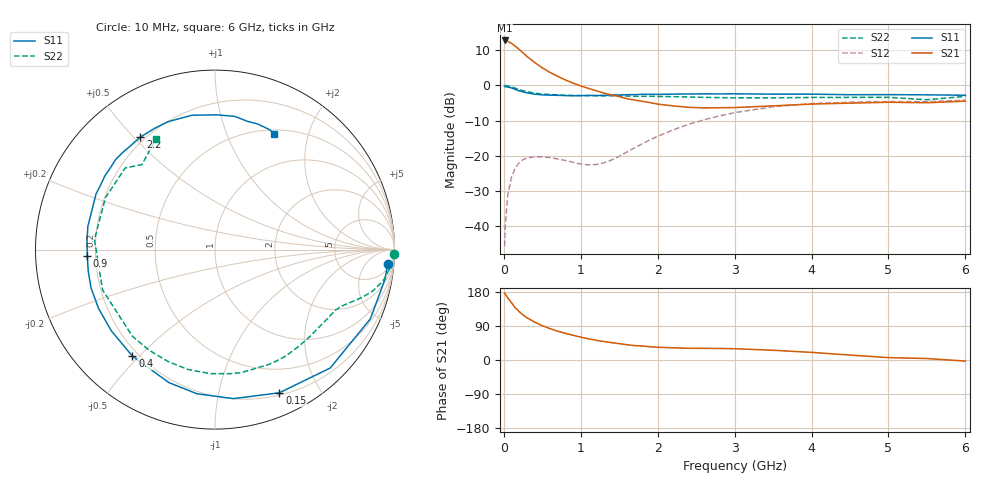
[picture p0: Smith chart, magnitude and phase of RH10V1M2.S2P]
! SIEMENS Small Signal Semiconductors
! BFR106
! Si NPN RF Bipolar Junction Transistor in SOT23
! VCE = 10 V  IC = 1.2 mA
! Common Emitter S-Parameters:  August  1996
# GHz  S  MA  R  50
!  f  S11  S21  S12  S22
! GHz  MAG  ANG  MAG  ANG  MAG  ANG  MAG  ANG
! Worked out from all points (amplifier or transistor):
!   36 points, 10 MHz to 6 GHz, reference 50 ohm
!   highest |S21| = 12.8 dB at 10 MHz (marker M1)
!   |S21| within 3 dB of that: start of sweep to 222.9 MHz
!   unconditionally stable (mu >= 1): 848.4 MHz to 1.802 GHz; 3.533 GHz to end of sweep
!   at 250 MHz: K = 0.27, MSG = 15.2 dB, |S12| = -21.1 dB
!   at 1.4 GHz: K = 1.32, MAG = 5.8 dB, |S12| = -21.2 dB
!   at 6 GHz: K = 1.02, MAG = -1.0 dB, |S12| = -4.2 dB
!   S11 on the Smith chart (normalised r, x): 10 MHz: 9, -21; 150 MHz: 0.22, -1.52; 400 MHz: 0.18, -0.48; 900 MHz: 0.17, -0.02; 2.2 GHz: 0.18, +0.52; 6 GHz: 0.55, +1.49
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0.01  0.9655 -4.7  4.348 176.3  0.0052 87.8  0.9989 -1.3
0.02  0.9616 -9.8  4.331 173.9  0.0107 87.4  0.9958 -2.3
0.05  0.9478 -24.0  4.227 164.1  0.0273 76.4  0.9836 -5.6
0.1  0.9205 -45.8  3.95 150.9  0.0501 65.1  0.9521 -10.6
0.15  0.8746 -65.8  3.583 137.5  0.0675 54.3  0.9113 -14.5
0.2  0.8367 -82.9  3.244 127.7  0.0798 46.7  0.8741 -17.1
0.25  0.8094 -97.2  2.893 118.5  0.088 39.8  0.8394 -19.4
0.3  0.7842 -109.1  2.577 111.6  0.093 35.2  0.814 -21.0
0.4  0.7509 -127.8  2.123 100.1  0.0968 28.0  0.7758 -23.8
0.5  0.7339 -141.9  1.775 90.5  0.0966 23.9  0.7529 -26.4
0.6  0.7269 -153.3  1.53 82.8  0.0942 21.6  0.742 -29.3
0.9  0.7126 -177.3  1.077 65.2  0.0808 26.3  0.7201 -38.6
1.1  0.72 169.7  0.907 56.0  0.0742 39.3  0.714 -45.8
1.6  0.7381 146.4  0.647 40.3  0.113 74.7  0.7062 -65.2
2.2  0.7521 123.5  0.511 32.1  0.2333 77.2  0.6916 -92.3
2.8  0.7565 104.7  0.481 30.5  0.3676 64.0  0.6702 -123.6
3.5  0.7509 89.3  0.512 25.7  0.497 45.4  0.6655 -160.3
4  0.7505 81.7  0.543 20.1  0.552 32.5  0.6739 175.2
4.5  0.7371 75.7  0.56 13.0  0.5779 21.3  0.6753 154.6
5  0.7391 71.2  0.576 6.3  0.5901 12.2  0.6762 137.7
5.5  0.7344 65.7  0.567 3.9  0.5872 7.7  0.6245 130.7
6  0.7243 62.9  0.597 -2.9  0.618 -0.5  0.6989 118.1
